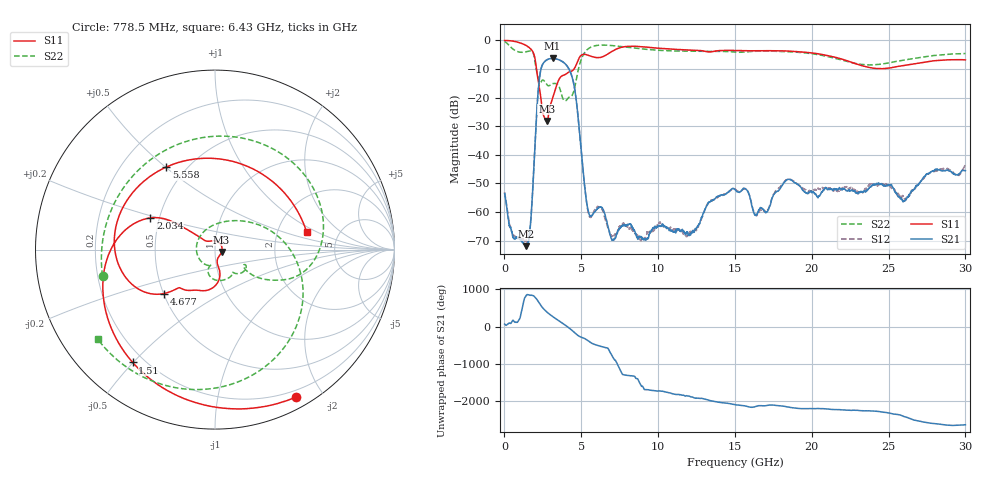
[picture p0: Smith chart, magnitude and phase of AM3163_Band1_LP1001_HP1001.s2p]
!Agilent Technologies,E8364B,MY43040894,A.07.50.67
!Agilent E8364B: A.07.50.67
!Date: Thursday, August 20, 2020 11:20:48
!Correction: S11(Full 2 Port(1,2))
!S21(Full 2 Port(1,2))
!S12(Full 2 Port(1,2))
!S22(Full 2 Port(1,2))
!S2P File: Measurements: S11, S21, S12, S22:
# Hz S  dB  R 50
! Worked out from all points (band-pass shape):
!   3201 points, 10 MHz to 30 GHz, reference 50 ohm
!   highest |S21| = -6.38 dB at 3.131 GHz (marker M1); lowest = -71.9 dB at 1.397 GHz (marker M2)
!   |S21| within 3 dB of the highest: 2.413 GHz to 4.124 GHz (1.711 GHz wide, 52.4 % of centre)
!   lowest |S11| = -28.2 dB at 2.747 GHz (marker M3), VSWR 1.08, Z = 53.8 - j1.38 ohm
!   |S11| at or under -10 dB: 2.082 GHz to 4.533 GHz (2.451 GHz wide, 74.1 % of centre)
!   |S22| runs from -21.2 to -0.5 dB; largest |S21 - S12| = 0.0042
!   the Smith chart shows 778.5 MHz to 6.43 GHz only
!   S11 on the Smith chart (normalised r, x): 778.5 MHz: 0.12, -1.69; 1.51 GHz: 0.16, -0.50; 2.034 GHz: 0.45, +0.19; 4.677 GHz: 0.50, -0.29; 5.558 GHz: 0.39, +0.50; 6.43 GHz: 2.92, +0.80
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1e7  -0.09 -5.3  -53.49 65.9  -53.09 -146.3  -0.46 -18.4
7.784938e8  -0.55 -61.1  -68.71 117.1  -68.79 -76.7  -3.83 -166.8
1.397038e9  -1.81 -114.7  -71.88 101.6  -69.85 11.7  -4.05 96.9
1.5095e9  -2.18 -126.1  -70.73 136.4  -70.14 126.2  -3.90 78.5
2.034325e9  -7.95 153.8  -31.38 51.9  -31.65 51.2  -9.13 -29.0
2.324853e9  -18.44 141.5  -11.50 -124.6  -11.50 -124.7  -14.78 -29.6
2.746588e9  -28.17 -19.1  -6.89 36.1  -6.90 36.0  -15.42 -50.4
3.130834e9  -20.36 -78.8  -6.38 -89.4  -6.39 -89.4  -15.16 -62.3
3.730634e9  -12.50 -105.1  -7.33 101.8  -7.33 102.0  -19.29 -109.1
4.677194e9  -8.51 -139.3  -21.10 154.0  -21.06 153.9  -13.69 51.2
5.014581e9  -5.20 -174.1  -39.63 68.8  -39.73 68.0  -6.46 -11.4
5.55815e9  -5.45 120.6  -61.20 -56.2  -61.64 -59.7  -2.62 -76.9
6.429734e9  -5.69 11.1  -59.20 168.8  -59.64 169.0  -1.70 -142.5
7.470012e9  -2.71 -106.5  -65.81 -29.7  -65.02 170.7  -2.13 163.5
8.472803e9  -2.11 178.6  -66.46 98.4  -67.23 -70.3  -2.75 120.6
1.000979e10  -2.80 99.7  -64.85 68.3  -63.80 65.7  -3.50 61.8
1.221218e10  -3.45 11.3  -66.91 -94.7  -67.01 94.8  -3.87 -14.1
1.5005e10  -3.57 -71.6  -52.11 57.0  -51.89 55.9  -4.13 -93.2
2.000958e10  -4.44 163.2  -53.19 -45.8  -52.56 -42.6  -4.71 137.0
2.276491e10  -8.04 60.0  -52.70 -92.1  -52.06 -109.5  -8.02 21.0
2.500479e10  -9.74 -62.4  -50.60 -165.9  -50.93 -168.4  -7.95 -92.0
3e10  -6.88 109.7  -45.56 -124.3  -43.54 -131.6  -4.65 103.2
